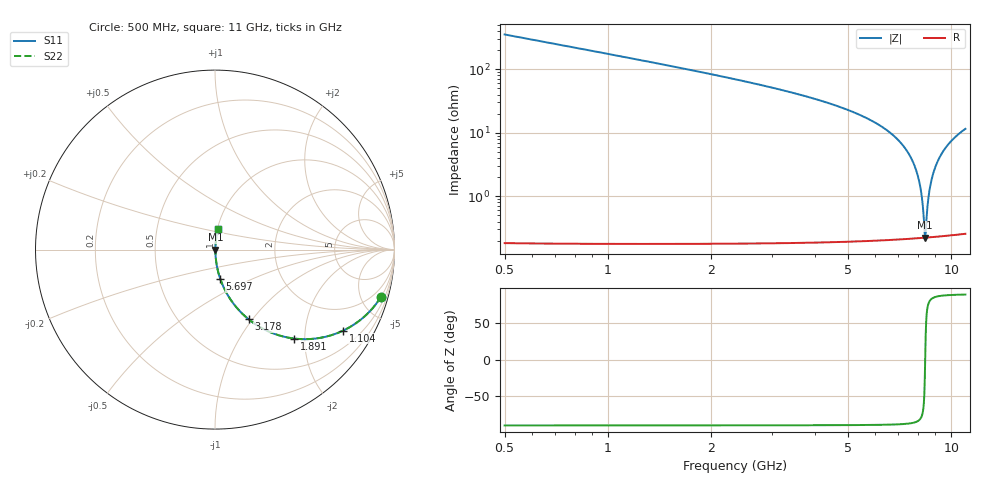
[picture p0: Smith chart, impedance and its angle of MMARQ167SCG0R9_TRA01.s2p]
! MMARQ167SCG0R9_TRA01  S-PARAMETER MODEL  ( General Type )
! Model Generated by TAIYO YUDEN Corporation (http://www.ty-top.com)
! Version 1.0
! TAIYO YUDEN Control No. 160201
! Copyright(c) 2016 TAIYO YUDEN CO.,LTD. All Rights Reserved.
! Product Description (link to TY-COMPAS)
! https://ds.yuden.co.jp/TYCOMPAS/or/detail?pn=MMARQ167SCG0R9BTRA01&u=M
! Products Name : Multilayer Ceramic Capacitors
! Characteristics :
!  Capacitance : 0.9 pF , Rated Voltage : 250V , TCC : CG / C0G
!  Case Size : 1.6 x 0.8 / 0.063 x 0.031 [mm/inch] , Thickness : 0.7 / 0.028 [mm/inch]
!  (Conditions: Temperature = 25 degC , DC Bias Current/Voltage = 0A / 0V)
! External Node Assignments :
!  1  o---| |---o  2
! GND o---------o GND
! Frequency Range : 500MHz  -  11000MHz  [ 401 STEP ]
# MHz S RI R 50
! Freq[MHz].  S11 Real  S11 Imag  S21 Real  S21 Imag  S12 Real  S12 Imag  S22 Real  S22 Imag
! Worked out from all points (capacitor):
!   401 points, 500 MHz to 11 GHz, reference 50 ohm
!   read as one part in series: C = 898 fF near 552.5 MHz
!   lowest |Z| = 223 mohm at 8.401 GHz (marker M1)
!   series resonance near 8.399 GHz, so ESL is about 400 pH
!   S11 on the Smith chart (normalised r, x): 500 MHz: 1.00, -7.06; 1.104 GHz: 1.00, -3.16; 1.891 GHz: 1.00, -1.78; 3.178 GHz: 1.00, -0.96; 5.697 GHz: 1.00, -0.34; 11 GHz: 1.01, +0.23
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500  0.9257 -0.262  0.0743 0.262  0.0743 0.262  0.9257 -0.262
1103.75  0.7132 -0.4517  0.2868 0.4517  0.2868 0.4517  0.7132 -0.4517
1891.25  0.4419 -0.4956  0.5581 0.4956  0.5581 0.4956  0.4419 -0.4956
2258.75  0.3467 -0.4747  0.6533 0.4747  0.6533 0.4747  0.3467 -0.4747
3177.5  0.1869 -0.3879  0.8131 0.3879  0.8131 0.3879  0.1869 -0.3879
4017.5  0.1051 -0.3039  0.8949 0.3039  0.8949 0.3039  0.1051 -0.3039
5697.5  0.0292 -0.1627  0.9708 0.1627  0.9708 0.1627  0.0292 -0.1627
5750  0.0279 -0.1589  0.9721 0.1589  0.9721 0.1589  0.0279 -0.1589
6800  0.01 -0.0887  0.99 0.0887  0.99 0.0887  0.01 -0.0887
7508.75  0.00435 -0.0471  0.9956 0.0471  0.9956 0.0471  0.00435 -0.0471
7850  0.00297 -0.0284  0.997 0.0284  0.997 0.0284  0.00297 -0.0284
8086.25  0.00244 -0.016  0.9976 0.016  0.9976 0.016  0.00244 -0.016
8217.5  0.00228 -0.0092  0.9977 0.0092  0.9977 0.0092  0.00228 -0.0092
8348.75  0.00222 -0.00254  0.9978 0.00254  0.9978 0.00254  0.00222 -0.00254
8401.25  0.00222 9.51e-05  0.9978 -9.51e-05  0.9978 -9.51e-05  0.00222 9.51e-05
8453.75  0.00223 0.00271  0.9978 -0.00271  0.9978 -0.00271  0.00223 0.00271
8585  0.00233 0.00918  0.9977 -0.00918  0.9977 -0.00918  0.00233 0.00918
8716.25  0.0025 0.0156  0.9975 -0.0156  0.9975 -0.0156  0.0025 0.0156
8952.5  0.003 0.0268  0.997 -0.0268  0.997 -0.0268  0.003 0.0268
9267.5  0.00404 0.0413  0.996 -0.0413  0.996 -0.0413  0.00404 0.0413
9976.25  0.00767 0.0722  0.9923 -0.0722  0.9923 -0.0722  0.00767 0.0722
11000  0.0156 0.1131  0.9844 -0.1131  0.9844 -0.1131  0.0156 0.1131
